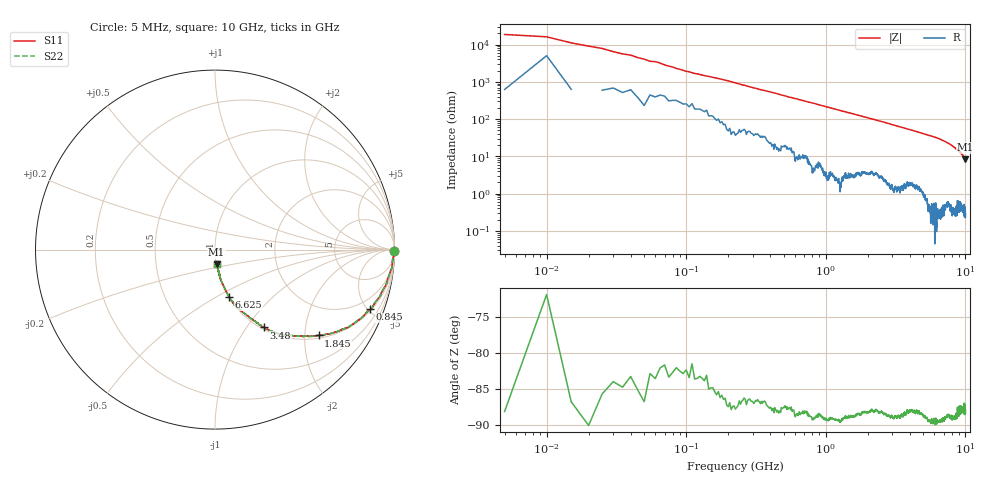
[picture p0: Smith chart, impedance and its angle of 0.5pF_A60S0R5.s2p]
! Amotech Co.,Ltd.
! http://www.amotech.co.kr/
! Part Number: A60S0R5
! These Parameters are Measured in Series Mode Connection
! Operation Temp=25[degC], DC Bias Voltage=0[V]
! Freq. Start=5[MHz] Stop=10[GHz], 2000[Steps]
! Date: Monday, July 13, 2020, 01:24:02
# GHZ S RI R 50.000000
!Freq.(Hz) S11(Real) S11(Imag) S21(Real) S21(Imag) S12(Real) S12(Imag) S22(Real) S22(Imag)
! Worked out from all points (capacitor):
!   2000 points, 5 MHz to 10 GHz, reference 50 ohm
!   read as one part in series: C = 818 fF near 55 MHz
!   lowest |Z| = 8.31 ohm at 9.995 GHz (marker M1)
!   S11 on the Smith chart (normalised r, x): 5 MHz: open; 845 MHz: 1.11, -5.15; 1.845 GHz: 1.07, -2.35; 3.48 GHz: 1.03, -1.21; 6.625 GHz: 1.01, -0.58; 10 GHz: 1.01, -0.17
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0.005  0.9998 -0.00535  0.000208 0.00535  0.000208 0.00535  0.9998 -0.00535
0.03  0.9981 -0.0153  0.00186 0.0153  0.00186 0.0153  0.9981 -0.0153
0.07  0.9937 -0.0343  0.00628 0.0343  0.00628 0.0343  0.9937 -0.0343
0.095  0.9916 -0.0479  0.00841 0.0479  0.00841 0.0479  0.9916 -0.0479
0.145  0.9889 -0.07  0.0111 0.07  0.0111 0.07  0.9889 -0.07
0.225  0.9847 -0.1045  0.0153 0.1045  0.0153 0.1045  0.9847 -0.1045
0.335  0.9668 -0.1529  0.0332 0.1529  0.0332 0.1529  0.9668 -0.1529
0.5  0.94 -0.2165  0.06 0.2165  0.06 0.2165  0.94 -0.2165
0.845  0.8639 -0.3323  0.1361 0.3323  0.1361 0.3323  0.8639 -0.3323
1.245  0.7485 -0.4284  0.2515 0.4284  0.2515 0.4284  0.7485 -0.4284
1.675  0.623 -0.4714  0.377 0.4714  0.377 0.4714  0.623 -0.4714
1.845  0.5773 -0.4784  0.4227 0.4784  0.4227 0.4784  0.5773 -0.4784
2.69  0.3912 -0.4752  0.6088 0.4752  0.6088 0.4752  0.3912 -0.4752
3.34  0.2891 -0.4423  0.7109 0.4423  0.7109 0.4423  0.2891 -0.4423
3.48  0.2728 -0.4335  0.7272 0.4335  0.7272 0.4335  0.2728 -0.4335
5.005  0.148 -0.3441  0.852 0.3441  0.852 0.3441  0.148 -0.3441
6.625  0.0788 -0.2646  0.9212 0.2646  0.9212 0.2646  0.0788 -0.2646
6.67  0.0769 -0.2624  0.9231 0.2624  0.9231 0.2624  0.0769 -0.2624
8.335  0.0323 -0.1692  0.9677 0.1692  0.9677 0.1692  0.0323 -0.1692
9.245  0.0194 -0.1227  0.9806 0.1227  0.9806 0.1227  0.0194 -0.1227
9.995  0.00906 -0.0821  0.9909 0.0821  0.9909 0.0821  0.00906 -0.0821
10  0.01 -0.0824  0.99 0.0824  0.99 0.0824  0.01 -0.0824
